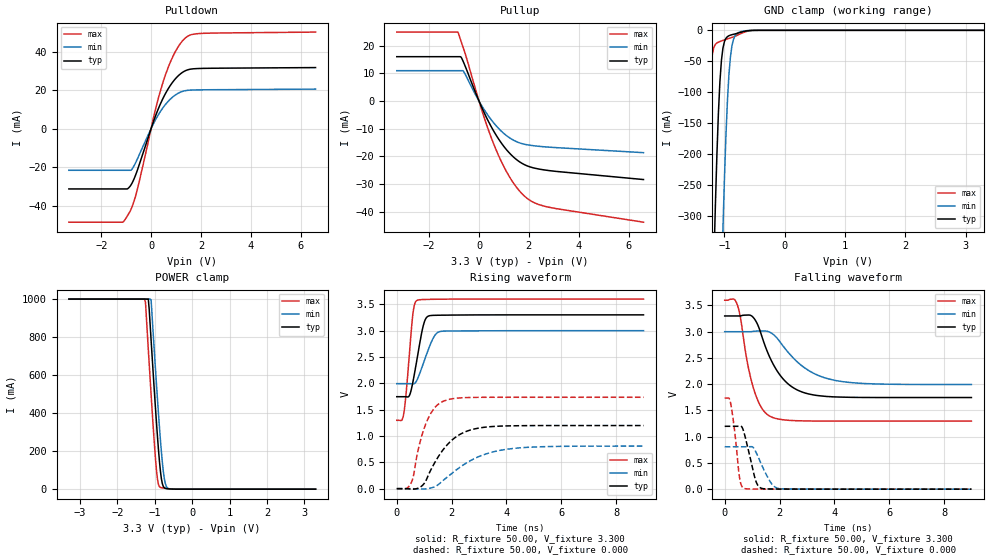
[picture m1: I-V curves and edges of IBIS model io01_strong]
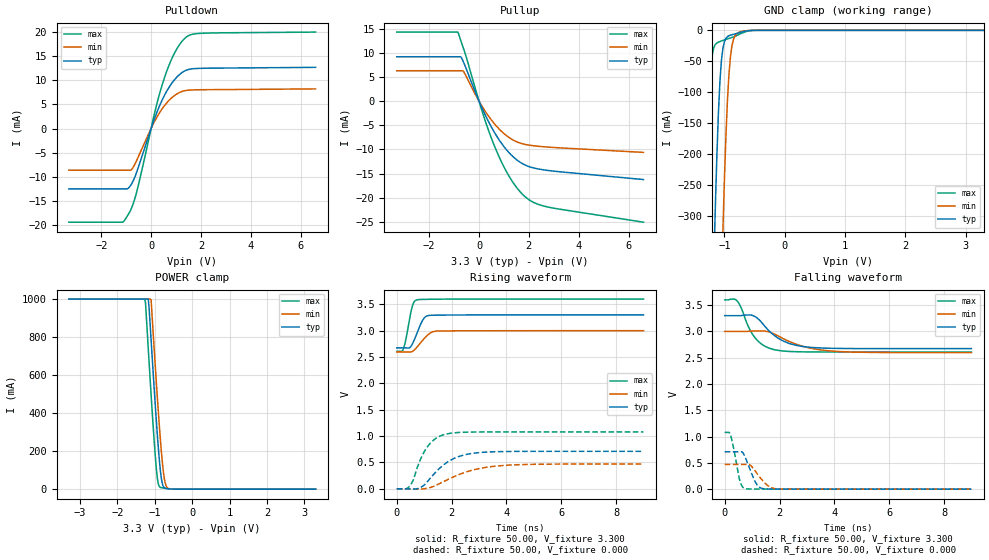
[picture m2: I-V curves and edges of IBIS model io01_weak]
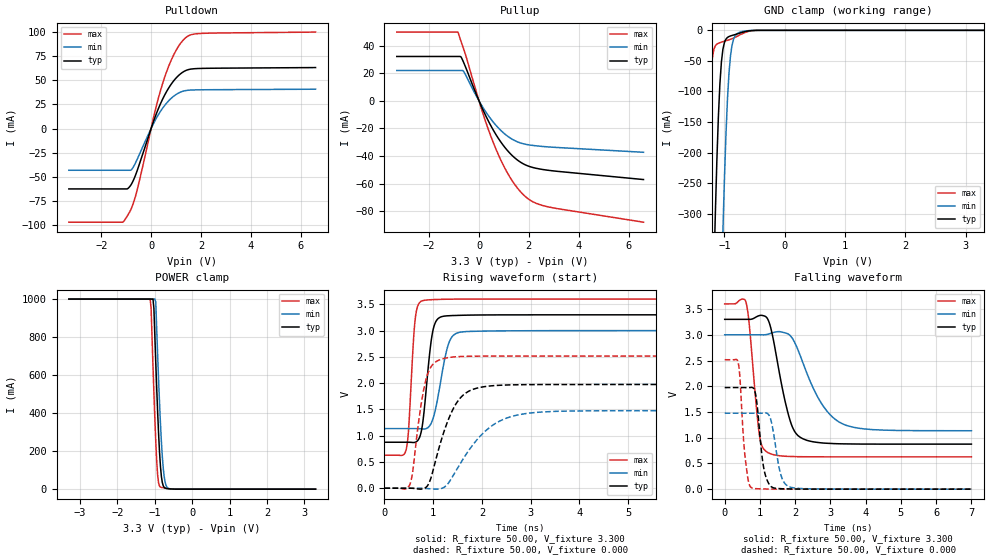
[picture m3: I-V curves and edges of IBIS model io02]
[IBIS Ver]   3.2
[File name]   rx63n_100tflga_065mm.ibs
[File Rev]   1.00
[Date]   May 21, 2013
[Source]   From silicon level SPICE model at
   Renesas Electronics Corporation
[Notes]
|   Renesas Microcomputer RX631/RX63N Group
|   RX631/RX63N 100pin TFLGA 0.65mm pitch
|   VCCQ : 3.30V
|(1) This IBIS file checked the format with ibischk5.
|   Format Error and Warning are 0.
|(2) Temperature described Tj.
|   Tj[deg]
|   Typical   45.0
|   Minimum   105.0
|   Maximum   -40.0
|(3) History
|   Rev 0.50  2012.09.10
|   New creation by Renesas Electronics Corporation
|   Rev 1.00  2013.05.21
|   Only change of revision number.
|   by Renesas Electronics Corporation
[Disclaimer]
   This information is for modeling purposes only,
   and is not guaranteed.
[Copyright]   Copyright 2012, Renesas Electronics Corporation ,
   All Rights Reserved
[Component]   rx63n_100tflga_065mm
[Manufacturer]  Renesas Electronics Corporation
[Package]
|   typ   min   max
R_pkg   310m   310m   310m
L_pkg   1.7nH   1.7nH   1.7nH
C_pkg   0.4pF   0.4pF   0.4pF
[Pin] signal_name   model_name
A1   P05   io02
A2   VREFH   POWER
A3   P07   io06
A4   VREFL0   GND
A5   P43   io14
A6   PD0   io01
A7   PD4   io01
A8   PE0   io01
A9   PE1   io01
A10   PE2   io01
B1   EMLE   input03
B2   AVSS0   GND
B3   AVCC0   POWER
B4   P40   io14
B5   P44   io14
B6   PD1   io01
B7   PD3   io01
B8   PD6   io01
B9   PD7   io01
B10   PE3   io01
C1   VCL   POWER
C2   VREFL   GND
C3   PJ3   io04
C4   VREFH0   POWER
C5   P42   io14
C6   P47   io14
C7   PD2   io01
C8   PD5   io01
C9   PE5   io01
C10   PE4   io01
D1   XCIN   NC
D2   XCOUT   NC
D3   MD   io04
D4   VBATT   POWER
D5   P45   io14
D6   P46   io14
D7   PE6   io01
D8   PE7   io01
D9   PA1   io07
D10   PA0   io07
E1   P37   io05
E2   VSS   GND
E3   RES#   input02
E4   P34   io04
E5   P41   io14
E6   PA2   io07
E7   PA6   io07
E8   PA4   io07
E9   PA5   io07
E10   PA3   io07
F1   P36   io03
F2   VCC   POWER
F3   P35   input01
F4   P32   io21
F5   P12   io18
F6   PB3   io07
F7   PB2   io07
F8   PB0   io07
F9   PA7   io07
F10   VSS   GND
G1   P33   io06
G2   P31   io21
G3   P30   io21
G4   P27   io07
G5   P53   io04
G6   P52   io07
G7   PB5   io07
G8   PB4   io07
G9   PB1   io07
G10   VCC   POWER
H1   P26   io07
H2   P25   io04
H3   P16   io15
H4   P15   io06
H5   P55   io07
H6   P54   io07
H7   PC7   io07
H8   PC6   io07
H9   PB6   io07
H10   PB7   io07
J1   P24   io04
J2   P21   io06
J3   P17   io15
J4   P13   io18
J5   VSS_USB   GND
J6   VCC_USB   POWER
J7   P50   io07
J8   PC4   io07
J9   PC0   io08
J10   PC1   io08
K1   P23   io04
K2   P22   io04
K3   P20   io06
K4   P14   io06
K5   USB0_DM   io09
K6   USB0_DP   io09
K7   P51   io07
K8   PC5   io07
K9   PC3   io08
K10   PC2   io08
[Diff Pin]   inv_pin   vdiff   tdelay_typ   tdelay_min   tdelay_max
K5   K6   0.000V   0.000s   NA   NA
[Model Selector]   io01
io01_strong   driver strength strong
io01_weak   driver strength weak
[Model Selector]   io07
io07_strong   driver strength strong
io07_weak   driver strength weak
[Model Selector]   io08
io08_strong   driver strength strong
io08_weak   driver strength weak
[Model Selector]   io15
io15a   driver strength strong
io15b   I2C buffer 1
[Model Selector]   io18
io18a   driver strength strong
io18b   I2C buffer 4
| Models and submodels in the file (21): io01_strong (I/O), io01_weak (I/O), io02 (I/O), io03 (I/O), io04 (I/O), io05 (I/O), io06 (I/O), io07_strong (I/O), io07_weak (I/O), io08_strong (I/O), io08_weak (I/O), io09 (I/O), io14 (I/O), io15a (I/O), io15b (I/O_open_drain), io18a (I/O), io18b (I/O_open_drain), io21 (I/O), input01 (Input), input02 (Input), input03 (Input)
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[Model]   io01_strong
Model_type   I/O
Polarity   Non-Inverting
Enable   Active-High
Vinl  =   0.660V
Vinh  =   2.640V
Vmeas =   1.650V
Cref  =   30.00pF
| variable   typ   min   max
C_comp   5.910pF   5.910pF   5.910pF
| variable   typ   min   max
[Temperature Range]   45.000   105.000   -40.000
| variable   typ   min   max
[Voltage Range]   3.300V   3.000V   3.600V
| variable   typ   min   max
[Pullup Reference]   3.300V   3.000V   3.600V
| variable   typ   min   max
[Pulldown Reference]   0.000V   0.000V   0.000V
| variable   typ   min   max
[POWER Clamp Reference] 3.300V   3.000V   3.600V
| variable   typ   min   max
[GND Clamp Reference]   0.000V   0.000V   0.000V
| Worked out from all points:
|   slope of the pulldown table from 0 to 0.495 V, typ, clamps not added: 30.7 ohm
|   slope of the pullup table from 0 to 0.495 V, typ, clamps not added: 52.9 ohm
|   GND clamp passes 1 mA (typ) near -0.63 V on its own axis
|   POWER clamp passes 1 mA (typ) near -0.58 V on its own axis
|   rising waveform, R_fixture 50.00, V_fixture 3.300: 20-80 % time 321ps typ, 432ps min, 222ps max; typ from 1.75 V to 3.3 V
|   rising waveform, R_fixture 50.00, V_fixture 0.000: 20-80 % time 961ps typ, 1.48ns min, 553ps max; typ from 0 V to 1.2 V
|   falling waveform, R_fixture 50.00, V_fixture 3.300: 20-80 % time 902ps typ, 1.27ns min, 542ps max; typ from 3.3 V to 1.75 V
|   falling waveform, R_fixture 50.00, V_fixture 0.000: 20-80 % time 324ps typ, 446ps min, 218ps max; typ from 1.2 V to 0 V
[Pulldown]
| io01_strong Pulldown rx631_rx63n
| Thu Mar 22 17:15:49 2012
| voltage   I(typ)   I(min)   I(max)
-3.3V     -31.31mA   -21.63mA   -48.57mA
-1.15V    -31.31mA   -21.63mA   -48.57mA
-1.025V   -31.31mA   -21.63mA   -46.81mA
-800mV    -29.1mA    -21.49mA   -41.71mA
-600mV    -23.34mA   -17.13mA   -33.95mA
175mV     6.49mA     4.538mA    9.911mA
525mV     16.92mA    11.68mA    25.93mA
950mV     25.49mA    17.23mA    39.38mA
1.4V      30.18mA    19.75mA    47.31mA
1.7V      31.04mA    20.05mA    49.02mA
2.1V      31.26mA    20.14mA    49.45mA
6.6V      31.67mA    20.5mA     50.09mA
[Pullup]
| io01_strong Pullup rx631_rx63n
| Thu Mar 22 17:15:49 2012
| voltage   I(typ)   I(min)   I(max)
-3.3V     16.04mA    10.98mA    24.94mA
-850mV    16.04mA    10.98mA    24.94mA
-725mV    15.94mA    10.98mA    21.66mA
-625mV    14.1mA     10.75mA    19.05mA
175mV     -3.59mA    -2.649mA   -5.083mA
700mV     -12.53mA   -9.072mA   -17.96mA
1V        -16.45mA   -11.75mA   -23.79mA
1.325V    -19.76mA   -13.87mA   -28.89mA
1.95V     -23.51mA   -15.85mA   -35.33mA
2.3V      -24.41mA   -16.28mA   -37.1mA
2.9V      -25.25mA   -16.74mA   -38.59mA
6.6V      -28.4mA    -18.67mA   -43.82mA
[GND Clamp]
| io01_strong GNDClamp rx631_rx63n
| Thu Mar 22 17:15:49 2012
| voltage   I(typ)   I(min)   I(max)
-3.3V     -1A        -1A        -1A
-1.325V   -1A        -1A        -369.2mA
-1.3V     -928.6mA   -1A        -269.7mA
-1.25V    -694.8mA   -1A        -112.6mA
-1.175V   -376mA     -953.3mA   -27.44mA
-1.15V    -283.8mA   -837.7mA   -22.69mA
-1.075V   -83.42mA   -512.2mA   -18.16mA
-1.025V   -28.94mA   -323mA     -16.39mA
-925mV    -8.707mA   -71.38mA   -13.1mA
-850mV    -6.468mA   -14.65mA   -10.64mA
-675mV    -1.81mA    -1.082mA   -3.186mA
3.3V      0A         0A         0A
[POWER Clamp]
| io01_strong PWRClamp rx631_rx63n
| Thu Mar 22 17:15:49 2012
| voltage   I(typ)   I(min)   I(max)
-3.3V     1A         1A         1A
-1.275V   1A         1A         1A
-1.25V    1A         1A         982.1mA
-1.175V   1A         1A         736.6mA
-1.1V     784.3mA    995.9mA    498mA
-1V       476.2mA    683.1mA    204.7mA
-950mV    332.1mA    533mA      87.52mA
-875mV    143.3mA    321.7mA    12.76mA
-825mV    55.42mA    197.2mA    7.873mA
-750mV    8.12mA     59.94mA    5.513mA
-625mV    1.619mA    2.607mA    2.132mA
3.3V      0A         0A         0A
[Ramp]
dV/dt_r   0.719/960.74p  0.485/1.48n   1.041/552.35p
dV/dt_f   0.933/901.13p  0.604/1.27n   1.382/541.71p
R_load = 50.00ohm
[Rising Waveform]
| io01_strong Rising-High rx631_rx63n
| Thu Mar 22 17:15:49 2012
R_fixture = 50.00
V_fixture = 3.300
V_fixture_min = 3.000
V_fixture_max = 3.600
C_fixture = 0.00pF
| Time   V(typ)   V(min)   V(max)
0s        1.746V     1.994V     1.297V
250ps     1.746V     1.994V     1.413V
450ps     1.759V     1.994V     2.489V
580ps     2.004V     1.989V     3.28V
645ps     2.183V     1.996V     3.491V
740ps     2.465V     2.064V     3.575V
1.045ns   3.216V     2.49V      3.592V
1.35ns    3.291V     2.878V     3.596V
1.585ns   3.293V     2.985V     3.598V
9ns       3.3V       3V         3.6V
[Rising Waveform]
| io01_strong Rising-Low rx631_rx63n
| Thu Mar 22 17:15:49 2012
R_fixture = 50.00
V_fixture = 0.000
C_fixture = 0.00pF
| Time   V(typ)   V(min)   V(max)
0s        0V         0V         0V
510ps     -7mV       0V         95mV
605ps     -9mV       -1mV       236mV
840ps     25mV       -7mV       868mV
1.075ns   164mV      -4mV       1.25V
1.385ns   494mV      37mV       1.537V
1.755ns   781mV      183mV      1.672V
2.55ns    1.09V      490mV      1.729V
3.975ns   1.191V     745mV      1.735V
9ns       1.198V     808mV      1.735V
[Falling Waveform]
| io01_strong Falling-High rx631_rx63n
| Thu Mar 22 17:15:49 2012
R_fixture = 50.00
V_fixture = 3.300
V_fixture_min = 3.000
V_fixture_max = 3.600
C_fixture = 0.00pF
| Time   V(typ)   V(min)   V(max)
0s        3.3V       3V         3.6V
445ps     3.3V       3V         3.533V
575ps     3.301V     3V         3.268V
825ps     3.317V     3V         2.418V
1.03ns    3.279V     3.006V     1.959V
1.325ns   2.961V     3.013V     1.567V
1.65ns    2.506V     2.99V      1.39V
2.46ns    1.947V     2.523V     1.308V
3.835ns   1.763V     2.095V     1.297V
9ns       1.746V     1.994V     1.297V
[Falling Waveform]
| io01_strong Falling-Low rx631_rx63n
| Thu Mar 22 17:15:49 2012
R_fixture = 50.00
V_fixture = 0.000
C_fixture = 0.00pF
| Time   V(typ)   V(min)   V(max)
0s        1.198V     808mV      1.735V
210ps     1.198V     808mV      1.65V
350ps     1.198V     808mV      1.163V
545ps     1.199V     808mV      210mV
710ps     1.068V     808mV      13mV
1.12ns    182mV      727mV      3mV
1.35ns    15mV       460mV      1mV
1.71ns    4mV        104mV      1mV
2.015ns   2mV        10mV       0V
9ns       0V         0V         0V
[Model]   io01_weak
Model_type   I/O
Polarity   Non-Inverting
Enable   Active-High
Vinl  =   0.660V
Vinh  =   2.640V
Vmeas =   1.650V
Cref  =   30.00pF
| variable   typ   min   max
C_comp   5.910pF   5.910pF   5.910pF
| variable   typ   min   max
[Temperature Range]   45.000   105.000   -40.000
| variable   typ   min   max
[Voltage Range]   3.300V   3.000V   3.600V
| variable   typ   min   max
[Pullup Reference]   3.300V   3.000V   3.600V
| variable   typ   min   max
[Pulldown Reference]   0.000V   0.000V   0.000V
| variable   typ   min   max
[POWER Clamp Reference] 3.300V   3.000V   3.600V
| variable   typ   min   max
[GND Clamp Reference]   0.000V   0.000V   0.000V
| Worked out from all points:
|   slope of the pulldown table from 0 to 0.495 V, typ, clamps not added: 76.6 ohm
|   slope of the pullup table from 0 to 0.495 V, typ, clamps not added: 92.4 ohm
|   GND clamp passes 1 mA (typ) near -0.63 V on its own axis
|   POWER clamp passes 1 mA (typ) near -0.58 V on its own axis
|   rising waveform, R_fixture 50.00, V_fixture 3.300: 20-80 % time 304ps typ, 415ps min, 218ps max; typ from 2.67 V to 3.3 V
|   rising waveform, R_fixture 50.00, V_fixture 0.000: 20-80 % time 931ps typ, 1.4ns min, 586ps max; typ from 0 V to 0.711 V
|   falling waveform, R_fixture 50.00, V_fixture 3.300: 20-80 % time 880ps typ, 1.24ns min, 596ps max; typ from 3.3 V to 2.67 V
|   falling waveform, R_fixture 50.00, V_fixture 0.000: 20-80 % time 333ps typ, 446ps min, 237ps max; typ from 0.711 V to 0 V
[Pulldown]
| io01_weak Pulldown rx631_rx63n
| Thu Mar 22 17:15:49 2012
| voltage   I(typ)   I(min)   I(max)
-3.3V     -12.52mA   -8.65mA    -19.43mA
-1.15V    -12.52mA   -8.65mA    -19.43mA
-1.025V   -12.52mA   -8.65mA    -18.72mA
-800mV    -11.64mA   -8.594mA   -16.68mA
-600mV    -9.336mA   -6.851mA   -13.58mA
175mV     2.596mA    1.815mA    3.964mA
525mV     6.766mA    4.671mA    10.37mA
950mV     10.19mA    6.891mA    15.75mA
1.4V      12.07mA    7.901mA    18.93mA
1.7V      12.42mA    8.02mA     19.61mA
2.1V      12.5mA     8.057mA    19.78mA
6.6V      12.7mA     8.228mA    20.01mA
[Pullup]
| io01_weak Pullup rx631_rx63n
| Thu Mar 22 17:15:49 2012
| voltage   I(typ)   I(min)   I(max)
-3.3V     9.166mA    6.276mA    14.26mA
-850mV    9.166mA    6.276mA    14.26mA
-725mV    9.114mA    6.276mA    12.4mA
-625mV    8.067mA    6.148mA    10.91mA
175mV     -2.054mA   -1.515mA   -2.91mA
700mV     -7.168mA   -5.188mA   -10.28mA
1.025V    -9.573mA   -6.827mA   -13.86mA
1.325V    -11.3mA    -7.926mA   -16.53mA
1.95V     -13.44mA   -9.058mA   -20.2mA
2.3V      -13.95mA   -9.303mA   -21.2mA
2.9V      -14.43mA   -9.565mA   -22.05mA
6.6V      -16.23mA   -10.61mA   -25.04mA
[GND Clamp]
| io01_weak GNDClamp rx631_rx63n
| Thu Mar 22 17:15:49 2012
| voltage   I(typ)   I(min)   I(max)
-3.3V     -1A        -1A        -1A
-1.325V   -1A        -1A        -369.2mA
-1.3V     -928.6mA   -1A        -269.7mA
-1.25V    -694.8mA   -1A        -112.6mA
-1.175V   -376mA     -953.3mA   -27.44mA
-1.15V    -283.8mA   -837.7mA   -22.69mA
-1.075V   -83.42mA   -512.2mA   -18.16mA
-1.025V   -28.94mA   -323mA     -16.39mA
-925mV    -8.707mA   -71.38mA   -13.1mA
-850mV    -6.468mA   -14.65mA   -10.64mA
-675mV    -1.81mA    -1.082mA   -3.186mA
3.3V      0A         0A         0A
[POWER Clamp]
| io01_weak PWRClamp rx631_rx63n
| Thu Mar 22 17:15:49 2012
| voltage   I(typ)   I(min)   I(max)
-3.3V     1A         1A         1A
-1.275V   1A         1A         1A
-1.25V    1A         1A         982.1mA
-1.175V   1A         1A         736.6mA
-1.1V     784.3mA    995.9mA    498mA
-1V       476.2mA    683.1mA    204.7mA
-950mV    332.1mA    533mA      87.52mA
-875mV    143.3mA    321.7mA    12.76mA
-825mV    55.42mA    197.2mA    7.873mA
-750mV    8.12mA     59.94mA    5.513mA
-625mV    1.619mA    2.607mA    2.132mA
3.3V      0A         0A         0A
[Ramp]
dV/dt_r   0.427/931.58p  0.283/1.40n   0.648/585.98p
dV/dt_f   0.376/877.26p  0.242/1.24n   0.595/596.02p
R_load = 50.00ohm
[Rising Waveform]
| io01_weak Rising-High rx631_rx63n
| Thu Mar 22 17:15:49 2012
R_fixture = 50.00
V_fixture = 3.300
V_fixture_min = 3.000
V_fixture_max = 3.600
C_fixture = 0.00pF
| Time   V(typ)   V(min)   V(max)
0s        2.673V     2.596V     2.608V
235ps     2.673V     2.596V     2.648V
330ps     2.674V     2.597V     2.833V
555ps     2.734V     2.602V     3.439V
630ps     2.816V     2.63V      3.544V
735ps     2.949V     2.688V     3.585V
985ps     3.229V     2.842V     3.594V
1.225ns   3.292V     2.956V     3.596V
1.57ns    3.295V     2.995V     3.598V
9ns       3.3V       3V         3.6V
[Rising Waveform]
| io01_weak Rising-Low rx631_rx63n
| Thu Mar 22 17:15:49 2012
R_fixture = 50.00
V_fixture = 0.000
C_fixture = 0.00pF
| Time   V(typ)   V(min)   V(max)
0s        0V         0V         0V
460ps     -2mV       0V         46mV
605ps     -6mV       -3mV       175mV
825ps     16mV       -4mV       509mV
1.12ns    136mV      12mV       800mV
1.435ns   324mV      67mV       960mV
1.815ns   495mV      164mV      1.039V
2.565ns   655mV      325mV      1.075V
3.875ns   707mV      442mV      1.079V
9ns       711mV      471mV      1.079V
[Falling Waveform]
| io01_weak Falling-High rx631_rx63n
| Thu Mar 22 17:15:49 2012
R_fixture = 50.00
V_fixture = 3.300
V_fixture_min = 3.000
V_fixture_max = 3.600
C_fixture = 0.00pF
| Time   V(typ)   V(min)   V(max)
0s        3.3V       3V         3.6V
350ps     3.3V       3V         3.615V
470ps     3.3V       3V         3.569V
865ps     3.312V     3.001V     3.09V
1.05ns    3.297V     3.008V     2.919V
1.4ns     3.137V     3.008V     2.739V
1.845ns   2.909V     2.942V     2.649V
2.61ns    2.735V     2.756V     2.614V
3.79ns    2.68V      2.632V     2.608V
9ns       2.673V     2.596V     2.608V
[Falling Waveform]
| io01_weak Falling-Low rx631_rx63n
| Thu Mar 22 17:15:49 2012
R_fixture = 50.00
V_fixture = 0.000
C_fixture = 0.00pF
| Time   V(typ)   V(min)   V(max)
0s        711mV      471mV      1.079V
205ps     711mV      471mV      1.037V
545ps     711mV      471mV      179mV
635ps     707mV      471mV      56mV
740ps     618mV      471mV      11mV
920ps     380mV      462mV      3mV
1.13ns    125mV      333mV      2mV
1.405ns   9mV        151mV      1mV
1.935ns   2mV        5mV        0V
9ns       0V         0V         0V
[Model]   io02
Model_type   I/O
Polarity   Non-Inverting
Enable   Active-High
Vinl  =   0.660V
Vinh  =   2.640V
Vmeas =   1.650V
Cref  =   30.00pF
| variable   typ   min   max
C_comp   4.810pF   4.810pF   4.810pF
| variable   typ   min   max
[Temperature Range]   45.000   105.000   -40.000
| variable   typ   min   max
[Voltage Range]   3.300V   3.000V   3.600V
| variable   typ   min   max
[Pullup Reference]   3.300V   3.000V   3.600V
| variable   typ   min   max
[Pulldown Reference]   0.000V   0.000V   0.000V
| variable   typ   min   max
[POWER Clamp Reference] 3.300V   3.000V   3.600V
| variable   typ   min   max
[GND Clamp Reference]   0.000V   0.000V   0.000V
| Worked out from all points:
|   slope of the pulldown table from 0 to 0.495 V, typ, clamps not added: 15.3 ohm
|   slope of the pullup table from 0 to 0.495 V, typ, clamps not added: 26.5 ohm
|   GND clamp passes 1 mA (typ) near -0.60 V on its own axis
|   POWER clamp passes 1 mA (typ) near -0.56 V on its own axis
|   rising waveform, R_fixture 50.00, V_fixture 3.300: 20-80 % time 160ps typ, 229ps min, 107ps max; typ from 0.875 V to 3.3 V
|   rising waveform, R_fixture 50.00, V_fixture 0.000: 20-80 % time 439ps typ, 750ps min, 233ps max; typ from 0 V to 1.97 V
|   falling waveform, R_fixture 50.00, V_fixture 3.300: 20-80 % time 438ps typ, 788ps min, 230ps max; typ from 3.3 V to 0.875 V
|   falling waveform, R_fixture 50.00, V_fixture 0.000: 20-80 % time 184ps typ, 224ps min, 154ps max; typ from 1.97 V to 0 V
[Pulldown]
| io02_strong Pulldown rx631_rx63n
| Thu Mar 22 17:15:49 2012
| voltage   I(typ)   I(min)   I(max)
-3.3V     -62.65mA   -43.27mA   -97.17mA
-1.15V    -62.65mA   -43.27mA   -97.17mA
-1.025V   -62.65mA   -43.27mA   -93.54mA
-800mV    -58.14mA   -42.96mA   -83.35mA
-600mV    -46.61mA   -34.21mA   -67.78mA
175mV     12.96mA    9.063mA    19.79mA
550mV     35.03mA    24.16mA    53.7mA
950mV     50.92mA    34.42mA    78.67mA
1.4V      60.32mA    39.47mA    94.54mA
1.7V      62.04mA    40.07mA    97.97mA
2.1V      62.48mA    40.25mA    98.84mA
6.6V      63.3mA     40.84mA    100.1mA
[Pullup]
| io02_strong Pullup rx631_rx63n
| Thu Mar 22 17:15:49 2012
| voltage   I(typ)   I(min)   I(max)
-3.3V     32.07mA    21.98mA    49.71mA
-850mV    32.07mA    21.98mA    49.71mA
-725mV    31.79mA    21.98mA    43.1mA
-625mV    28.07mA    21.44mA    37.9mA
150mV     -6.167mA   -4.559mA   -8.713mA
675mV     -24.26mA   -17.6mA    -34.7mA
975mV     -32.23mA   -23.07mA   -46.52mA
1.3V      -39mA      -27.43mA   -56.92mA
1.925V    -46.81mA   -31.61mA   -70.21mA
2.3V      -48.81mA   -32.55mA   -74.14mA
2.8V      -50.28mA   -33.35mA   -76.77mA
6.6V      -56.92mA   -37.21mA   -87.76mA
[GND Clamp]
| io02_strong GNDClamp rx631_rx63n
| Thu Mar 22 17:15:49 2012
| voltage   I(typ)   I(min)   I(max)
-3.3V     -1A        -1A        -1A
-1.325V   -1A        -1A        -406.6mA
-1.3V     -983.2mA   -1A        -299.4mA
-1.225V   -615mA     -1A        -75.45mA
-1.175V   -395.1mA   -992.5mA   -30.98mA
-1.15V    -297.6mA   -869.7mA   -25.1mA
-1.075V   -87.49mA   -526mA     -20.19mA
-1.025V   -30.91mA   -328.2mA   -18.56mA
-925mV    -10.2mA    -71.04mA   -15.59mA
-850mV    -7.712mA   -14.99mA   -12.74mA
-675mV    -2.503mA   -1.438mA   -4.223mA
3.3V      0A         0A         0A
[POWER Clamp]
| io02_strong PWRClamp rx631_rx63n
| Thu Mar 22 17:15:49 2012
| voltage   I(typ)   I(min)   I(max)
-3.3V     1A         1A         1A
-1.125V   1A         1A         1A
-1.1V     1A         1A         952.1mA
-1.05V    1A         1A         650.2mA
-1.025V   951.6mA    1A         507.1mA
-975mV    665.2mA    983.6mA    250.2mA
-925mV    406mA      705.8mA    73.52mA
-850mV    120.7mA    345.8mA    11.13mA
-800mV    34.79mA    171.7mA    8.224mA
-750mV    9.544mA    66.61mA    6.556mA
-625mV    2.042mA    3.124mA    2.737mA
3.3V      0A         0A         0A
[Ramp]
dV/dt_r   1.184/438.21p  0.886/749.00p  1.509/232.71p
dV/dt_f   1.455/438.02p  1.119/787.01p  1.783/229.46p
R_load = 50.00ohm
[Rising Waveform]
| io02_strong Rising-High rx631_rx63n
| Thu Mar 22 17:15:49 2012
R_fixture = 50.00
V_fixture = 3.300
V_fixture_min = 3.000
V_fixture_max = 3.600
C_fixture = 0.00pF
| Time   V(typ)   V(min)   V(max)
0s        875mV      1.135V     628mV
445ps     876mV      1.135V     734mV
495ps     875mV      1.135V     1.111V
625ps     873mV      1.135V     3.163V
760ps     1.097V     1.13V      3.561V
975ps     2.901V     1.27V      3.589V
1.16ns    3.261V     2.067V     3.595V
1.345ns   3.284V     2.816V     3.598V
1.575ns   3.291V     2.973V     3.599V
7ns       3.3V       3V         3.6V
[Rising Waveform]
| io02_strong Rising-Low rx631_rx63n
| Thu Mar 22 17:15:49 2012
R_fixture = 50.00
V_fixture = 0.000
C_fixture = 0.00pF
| Time   V(typ)   V(min)   V(max)
0s        0V         0V         0V
520ps     0V         0V         67mV
840ps     9mV        -4mV       2.022V
965ps     227mV      -13mV      2.324V
1.155ns   880mV      -9mV       2.452V
1.39ns    1.472V     210mV      2.496V
1.65ns    1.799V     608mV      2.51V
2.09ns    1.938V     1.104V     2.515V
2.6ns     1.967V     1.363V     2.515V
7ns       1.974V     1.476V     2.515V
[Falling Waveform]
| io02_strong Falling-High rx631_rx63n
| Thu Mar 22 17:15:49 2012
R_fixture = 50.00
V_fixture = 3.300
V_fixture_min = 3.000
V_fixture_max = 3.600
C_fixture = 0.00pF
| Time   V(typ)   V(min)   V(max)
0s        3.3V       3V         3.6V
610ps     3.3V       3V         3.618V
700ps     3.299V     3V         3.177V
985ps     3.373V     3V         1.049V
1.205ns   3.323V     3.007V     719mV
1.815ns   1.429V     3.009V     637mV
2.145ns   1.007V     2.591V     631mV
2.74ns    900mV      1.672V     629mV
3.33ns    881mV      1.274V     628mV
7ns       875mV      1.135V     628mV
[Falling Waveform]
| io02_strong Falling-Low rx631_rx63n
| Thu Mar 22 17:15:49 2012
R_fixture = 50.00
V_fixture = 0.000
C_fixture = 0.00pF
| Time   V(typ)   V(min)   V(max)
0s        1.974V     1.476V     2.515V
385ps     1.974V     1.476V     2.454V
570ps     1.974V     1.476V     683mV
755ps     1.978V     1.476V     29mV
890ps     1.793V     1.476V     10mV
1.125ns   352mV      1.48V      4mV
1.36ns    32mV       1.19V      2mV
1.61ns    9mV        242mV      1mV
1.88ns    4mV        36mV       0V
7ns       0V         0V         0V
